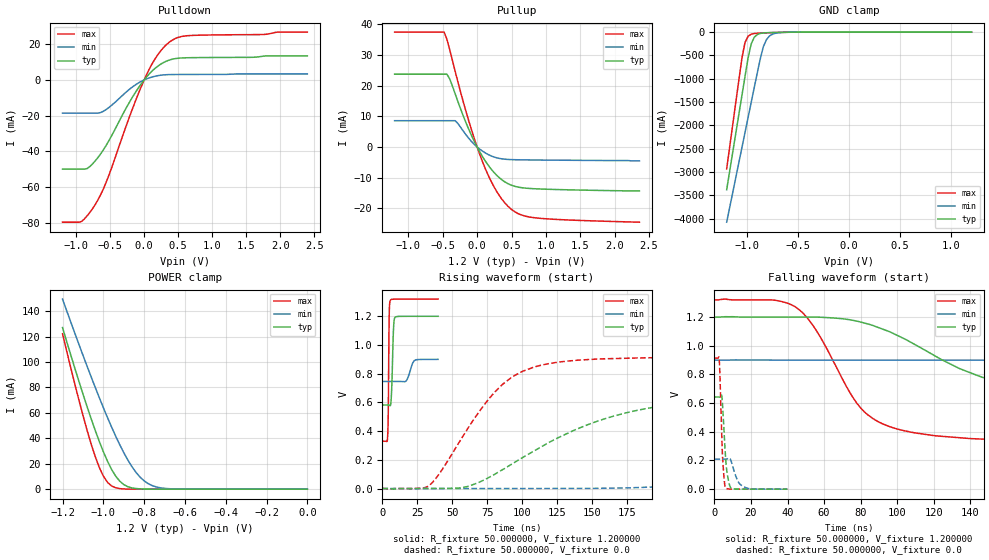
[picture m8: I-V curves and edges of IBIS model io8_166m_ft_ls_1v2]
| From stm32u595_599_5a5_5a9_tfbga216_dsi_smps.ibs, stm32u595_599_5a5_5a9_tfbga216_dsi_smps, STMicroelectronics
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|   Model io8_166m_ft_ls_1v2
[Model]  io8_166m_ft_ls_1v2
Model_type I/O
Polarity   Non-Inverting
Enable   Active-Low
Vinl =   0.360000V
Vinh =   0.840000V
Vmeas =  0.600000V
Cref =   50.000000pF
Rref =   100.000000M
Vref =   0.0V
C_comp   3.151400pF   3.086700pF   3.197700pF
[Temperature Range]   25.000000   0.140000k   -40.000000
[Pullup Reference]   1.200000V   0.900000V   1.320000V
[Pulldown Reference]   0.0V   0.0V   0.0V
[POWER Clamp Reference]   1.200000V   0.900000V   1.320000V
[GND Clamp Reference]   0.0V   0.0V   0.0V
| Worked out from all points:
|   slope of the pulldown table from 0 to 0.18 V, typ, clamps not added: 25.4 ohm
|   slope of the pullup table from 0 to 0.18 V, typ, clamps not added: 27.8 ohm
|   GND clamp passes 1 mA (typ) near -0.51 V on its own axis
|   POWER clamp passes 1 mA (typ) near -0.86 V on its own axis
|   rising waveform, R_fixture 50.000000, V_fixture 1.200000: 20-80 % time 1.12ns typ, 3.03ns min, 551ps max; typ from 0.582 V to 1.2 V
|   rising waveform, R_fixture 50.000000, V_fixture 0.0: 20-80 % time 83.8ns typ, 204ns min, 40.6ns max; typ from 0 V to 0.643 V
|   falling waveform, R_fixture 50.000000, V_fixture 1.200000: 20-80 % time 70.8ns typ, 188ns min, 28.1ns max; typ from 1.2 V to 0.582 V
|   falling waveform, R_fixture 50.000000, V_fixture 0.0: 20-80 % time 1.99ns typ, 3.7ns min, 1.49ns max; typ from 0.643 V to 0 V
[Pulldown]
|Voltage   I(typ)   I(min)   I(max)
-1.2V     -49.86mA   -18.57mA   -79.57mA
-920mV    -49.86mA   -18.57mA   -79.2mA
-840mV    -49.6mA    -18.57mA   -76.08mA
-720mV    -45.32mA   -18.57mA   -69.74mA
-560mV    -36.71mA   -16.58mA   -57.44mA
-200mV    -11.43mA   -4.74mA    -19.03mA
0V        0A         -500fA     0A
160mV     6.477mA    2.075mA    11.78mA
360mV     10.99mA    2.989mA    20.81mA
480mV     12.07mA    3.054mA    23.53mA
640mV     12.43mA    3.074mA    24.76mA
2.4V      13.46mA    3.369mA    26.78mA
[Pullup]
|Voltage   I(typ)   I(min)   I(max)
-1.2V     23.71mA    8.575mA    37.42mA
-480mV    23.71mA    8.575mA    37.42mA
-440mV    23.71mA    8.575mA    35.15mA
-400mV    22.24mA    8.575mA    31.81mA
-320mV    17.36mA    8.575mA    24.69mA
-120mV    5.681mA    2.787mA    8.394mA
80mV      -3.179mA   -1.366mA   -4.88mA
280mV     -9.096mA   -3.479mA   -14.29mA
520mV     -12.61mA   -4.111mA   -20.65mA
680mV     -13.33mA   -4.182mA   -22.38mA
920mV     -13.66mA   -4.239mA   -23.22mA
2.36V     -14.3mA    -4.5mA     -24.47mA
[GND_clamp]
|Voltage   I(typ)   I(min)   I(max)
-1.2V     -3.379A    -4.076A    -2.932A
-1.05V    -1.35A     -2.47A     -550.7mA
-1.02V    -947.8mA   -2.149A    -221.5mA
-990mV    -552.4mA   -1.829A    -88.44mA
-960mV    -255.3mA   -1.51A     -44.87mA
-930mV    -111.8mA   -1.191A    -30.68mA
-870mV    -28.36mA   -564.6mA   -21.34mA
-840mV    -18.65mA   -309.5mA   -18.49mA
-810mV    -14.07mA   -161.6mA   -15.92mA
-780mV    -11.37mA   -83.33mA   -13.53mA
-600mV    -3.009mA   -4.322mA   -3.091mA
1.2V      0A         13.65nA    0A
[POWER_clamp]
|Voltage   I(typ)   I(min)   I(max)
-1.2V     127mA      149.4mA    122.2mA
-1.12V    84.97mA    114mA      70.27mA
-1.06V    55.51mA    88.42mA    35.67mA
-1.02V    37.63mA    72.04mA    17.17mA
-1V       29.51mA    64.13mA    10.3mA
-960mV    15.69mA    48.99mA    2.571mA
-900mV    3.624mA    28.77mA    182.8uA
-840mV    490.7uA    13.24mA    11.35uA
-800mV    116.8uA    6.532mA    1.77uA
-740mV    13.2uA     1.724mA    109.1nA
-620mV    167.4nA    79.36uA    0A
0V        0A         17.87nA    0A
[Ramp]
| variable   typ   min   max
dV/dt_r  0.38562/83.72421n   0.12523/0.20346u   0.54824/40.54228n
dV/dt_f  0.37086/70.72236n   92.18400m/0.18810u  0.59438/28.02457n
R_load = 50.000000
[Rising Waveform]
R_fixture= 50.000000
V_fixture= 1.200000
V_fixture_min= 0.900000
V_fixture_max= 1.320000
|time   V(typ)   V(min)   V(max)
0s        581.9mV    745.9mV    329.4mV
3.764ns   582mV      745.9mV    360.7mV
4.244ns   582mV      745.9mV    539.7mV
4.885ns   580.5mV    745.9mV    1.194V
5.606ns   577.3mV    745.9mV    1.308V
6.486ns   653.6mV    745.9mV    1.317V
7.848ns   1.081V     745.9mV    1.319V
8.809ns   1.189V     745.9mV    1.319V
22.82ns   1.2V       891.3mV    1.32V
39.88ns   1.2V       900mV      1.32V
[Rising Waveform]
R_fixture= 50.000000
V_fixture= 0.0
V_fixture_min= 0.0
V_fixture_max= 0.0
|time   V(typ)   V(min)   V(max)
0s        1.999nV    239.2nV    1.184nV
34.03ns   -72.53uV   -36.45uV   24.96mV
60.06ns   11.91mV    -31.29uV   401.4mV
86.09ns   131.6mV    31.27uV    725.6mV
108.1ns   259mV      144.5uV    844.3mV
132.1ns   382.5mV    542.8uV    887.5mV
198.2ns   572.2mV    12.12mV    911.4mV
298.3ns   634.7mV    80.39mV    913.6mV
516.5ns   642.8mV    185.1mV    913.7mV
997ns     642.7mV    209.2mV    913.8mV
[Falling Waveform]
R_fixture= 50.000000
V_fixture= 1.200000
V_fixture_min= 0.900000
V_fixture_max= 1.320000
|time   V(typ)   V(min)   V(max)
0s        1.2V       900mV      1.32V
44.04ns   1.2V       900mV      1.273V
54.05ns   1.2V       900mV      1.139V
84.08ns   1.152V     900mV      516.4mV
104.1ns   1.047V     900mV      406.7mV
140.1ns   811mV      899.8mV    352.6mV
198.2ns   654.8mV    896.1mV    333.4mV
298.3ns   594mV      850.4mV    329.6mV
494.5ns   582.2mV    768.2mV    329.4mV
997ns     581.9mV    745.9mV    329.4mV
[Falling Waveform]
R_fixture= 50.000000
V_fixture= 0.0
V_fixture_min= 0.0
V_fixture_max= 0.0
|time   V(typ)   V(min)   V(max)
0s        642.7mV    209.2mV    913.8mV
2.563ns   642.7mV    209.3mV    909.7mV
3.924ns   656.4mV    209.3mV    410.3mV
4.404ns   591.5mV    209.3mV    235.3mV
6.006ns   239.4mV    208.9mV    11mV
6.967ns   109.2mV    211mV      3.239mV
9.049ns   6.07mV     198.6mV    569.1uV
12.65ns   632.7uV    60.35mV    -12.9uV
16.1ns    83.55uV    16.78mV    -63.55uV
39.88ns   1.999nV    239.2nV    1.184nV
